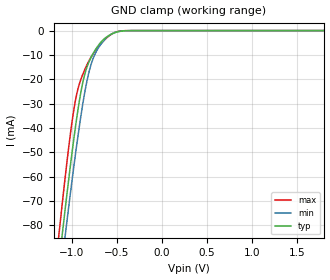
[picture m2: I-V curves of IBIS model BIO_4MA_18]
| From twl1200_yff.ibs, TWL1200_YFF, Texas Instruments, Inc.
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[Model]   BIO_4MA_18
Model_type  Input
Vinl=0.63
Vinh=1.17
| variable   typ   min   max
C_comp   2.87pF   2.44pF   3.48pF
[Temperature Range]   40   100   -40
| Ambient temperature   25   85   -40
[Voltage range]   1.8   1.65   1.95
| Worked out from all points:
|   GND clamp passes 1 mA (typ) near -0.53 V on its own axis
[GND Clamp]
| BIO_4MA_18
|   Voltage   I(typ)   I(min)   I(max)
-1.8V     -328.7mA   -328.2mA   -331mA
-1.145V   -97.37mA   -107.5mA   -85.45mA
-1.13V    -92.43mA   -102.7mA   -80.25mA
-1.095V   -81.06mA   -91.79mA   -68.33mA
-1.065V   -71.51mA   -82.55mA   -58.45mA
-960mV    -40.49mA   -51.77mA   -29.36mA
-860mV    -18.95mA   -26.82mA   -16.62mA
-810mV    -13.18mA   -17.59mA   -12.65mA
-755mV    -9.083mA   -10.95mA   -9.266mA
-585mV    -2.026mA   -2.094mA   -2.223mA
-400mV    -76.72uA   -76.15uA   -35.92uA
1.8V      454.1pA    57.07nA    58.32pA
